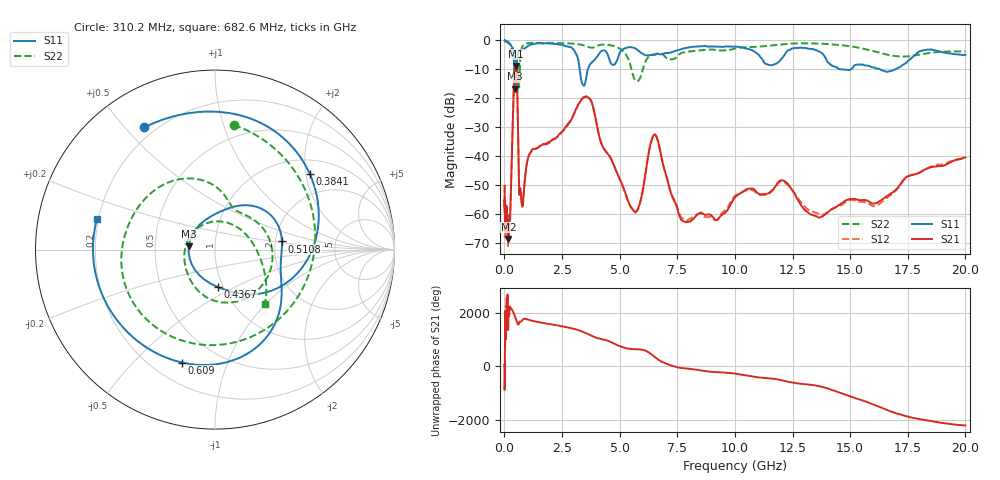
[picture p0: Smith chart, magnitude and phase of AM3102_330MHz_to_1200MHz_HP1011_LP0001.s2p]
! Date/Time: Tue, Sep 11, 2018 5:19 PM
! Network Analyzer: Agilent Technologies E8362B Rev: A.07.50.63
! Sweep from 0.010 to 20.000 GHz, 1601 Points, Sweep Type: LOG
! Power Supply: 4.949 V, 0.001 A
# Hz S DB R 50
!freq MagS11 AngS11 MagS21 AngS21 MagS12 AngS12 MagS22 AngS22
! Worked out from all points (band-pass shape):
!   1601 points, 10 MHz to 20 GHz, reference 50 ohm
!   highest |S21| = -8.83 dB at 482.5 MHz (marker M1); lowest = -68.5 dB at 174.6 MHz (marker M2)
!   |S21| within 3 dB of the highest: 429.5 MHz to 539.2 MHz (109.7 MHz wide, 22.7 % of centre)
!   lowest |S11| = -16.6 dB at 453.6 MHz (marker M3), VSWR 1.35, Z = 37.2 + j1.46 ohm
!   |S11| at or under -10 dB: 3.266 GHz to 3.622 GHz (355.8 MHz wide, 10.3 % of centre); 14.63 GHz to 15.03 GHz (392.1 MHz wide, 2.64 % of centre); 16.3 GHz to 16.95 GHz (648.4 MHz wide, 3.9 % of centre)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
!   |S22| runs from -16.2 to -0.2 dB; largest |S21 - S12| = 0.0053
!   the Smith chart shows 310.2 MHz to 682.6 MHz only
!   S11 on the Smith chart (normalised r, x): 310.2 MHz: 0.16, +0.57; 384.1 MHz: 1.36, +2.11; 436.7 MHz: 0.95, -0.41; 510.8 MHz: 2.17, +0.23; 609 MHz: 0.32, -0.70; 682.6 MHz: 0.19, +0.12
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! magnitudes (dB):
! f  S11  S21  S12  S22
! 10 MHz  0.0  -50.2  -50.0  -0.2
! 35.55 MHz  0.0  -64.5  -61.5  -0.3
! 126.4 MHz  -0.4  -64.6  -63.8  -0.7
! 174.6 MHz  -0.7  -68.5  -67.0  -0.9
! 252.9 MHz  -1.3  -60.5  -59.3  -1.7
! 310.2 MHz  -2.1  -43.9  -43.9  -3.1
! 384.1 MHz  -3.4  -21.6  -21.6  -5.6
! 436.7 MHz  -13.6  -10.9  -10.9  -5.6
! 447.2 MHz  -16.3  -9.9  -9.9  -5.9
! 453.6 MHz  -16.6  -9.4  -9.5  -6.0
! 482.5 MHz  -9.9  -8.8  -8.9  -6.8
! 510.8 MHz  -8.5  -9.2  -9.2  -9.6
! 609 MHz  -3.7  -39.9  -40.0  -12.0
! 682.6 MHz  -3.3  -51.1  -51.2  -7.7
! 1.59 GHz  -1.0  -36.3  -36.3  -0.8
! 3.617 GHz  -10.1  -19.6  -19.4  -2.2
! 5.652 GHz  -2.7  -59.1  -59.4  -13.5
! 6.487 GHz  -5.0  -32.6  -32.9  -4.8
! 7.92 GHz  -2.5  -62.7  -62.1  -3.9
! 12.03 GHz  -6.2  -48.3  -48.7  -1.4
! 13.74 GHz  -4.2  -60.9  -60.4  -1.1
! 20 GHz  -5.0  -40.4  -40.9  -3.8
